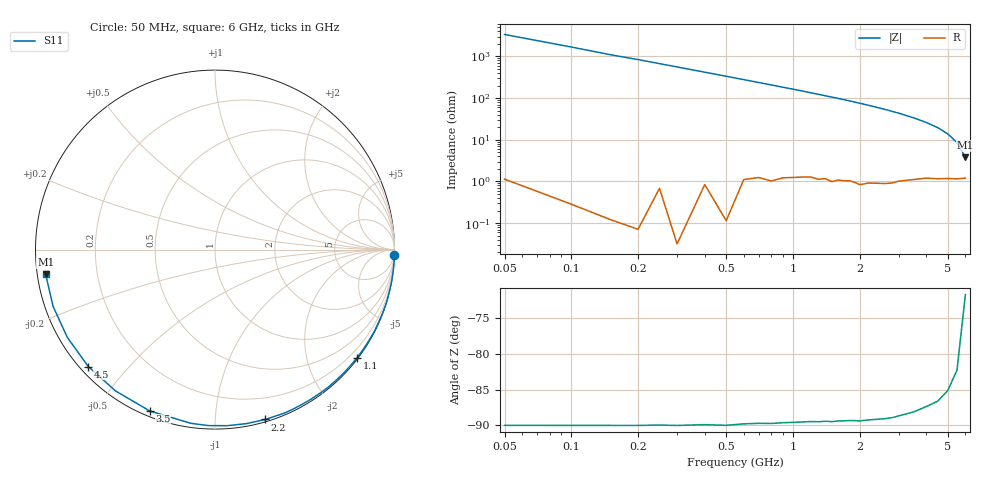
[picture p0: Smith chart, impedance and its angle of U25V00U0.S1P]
! SIEMENS Discrete & RF Semiconductors
! BBY52-02W
! Si Tuning Diode in SCD-80
! VR = 5 V
! S-Parameters:  September  1997
# GHz  S  MA  R  50
!  f  S11
! GHz  MAG  ANG
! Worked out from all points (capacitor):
!   34 points, 50 MHz to 6 GHz, reference 50 ohm
!   read as one part to ground: C = 945 fF near 50 MHz
!   lowest |Z| = 3.82 ohm at 6 GHz (marker M1)
!   S11 on the Smith chart (normalised r, x): 50 MHz: 0, -67; 1.1 GHz: 0.03, -2.96; 2.2 GHz: 0.02, -1.34; 3.5 GHz: 0.02, -0.67; 4.5 GHz: 0.02, -0.39; 6 GHz: 0.02, -0.07
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0.05  1 -1.7
0.15  1 -5.2
0.2  1 -6.8
0.3  1 -10.2
0.4  0.9995 -13.6
0.5  0.9999 -17.0
0.6  0.9986 -20.4
0.8  0.9977 -27.2
1  0.9958 -33.9
1.1  0.9948 -37.3
1.3  0.9937 -44.0
1.4  0.9925 -47.4
1.5  0.9928 -50.7
1.6  0.9911 -53.9
1.7  0.9905 -57.2
1.9  0.9894 -63.8
2  0.9898 -67.0
2.2  0.987 -73.5
2.4  0.9852 -79.8
2.6  0.9835 -86.0
2.8  0.9812 -92.1
3  0.9771 -97.9
3.5  0.9699 -112.0
4  0.9628 -125.1
4.5  0.9606 -137.3
5  0.9571 -149.2
5.5  0.956 -160.7
6  0.9534 -171.7
